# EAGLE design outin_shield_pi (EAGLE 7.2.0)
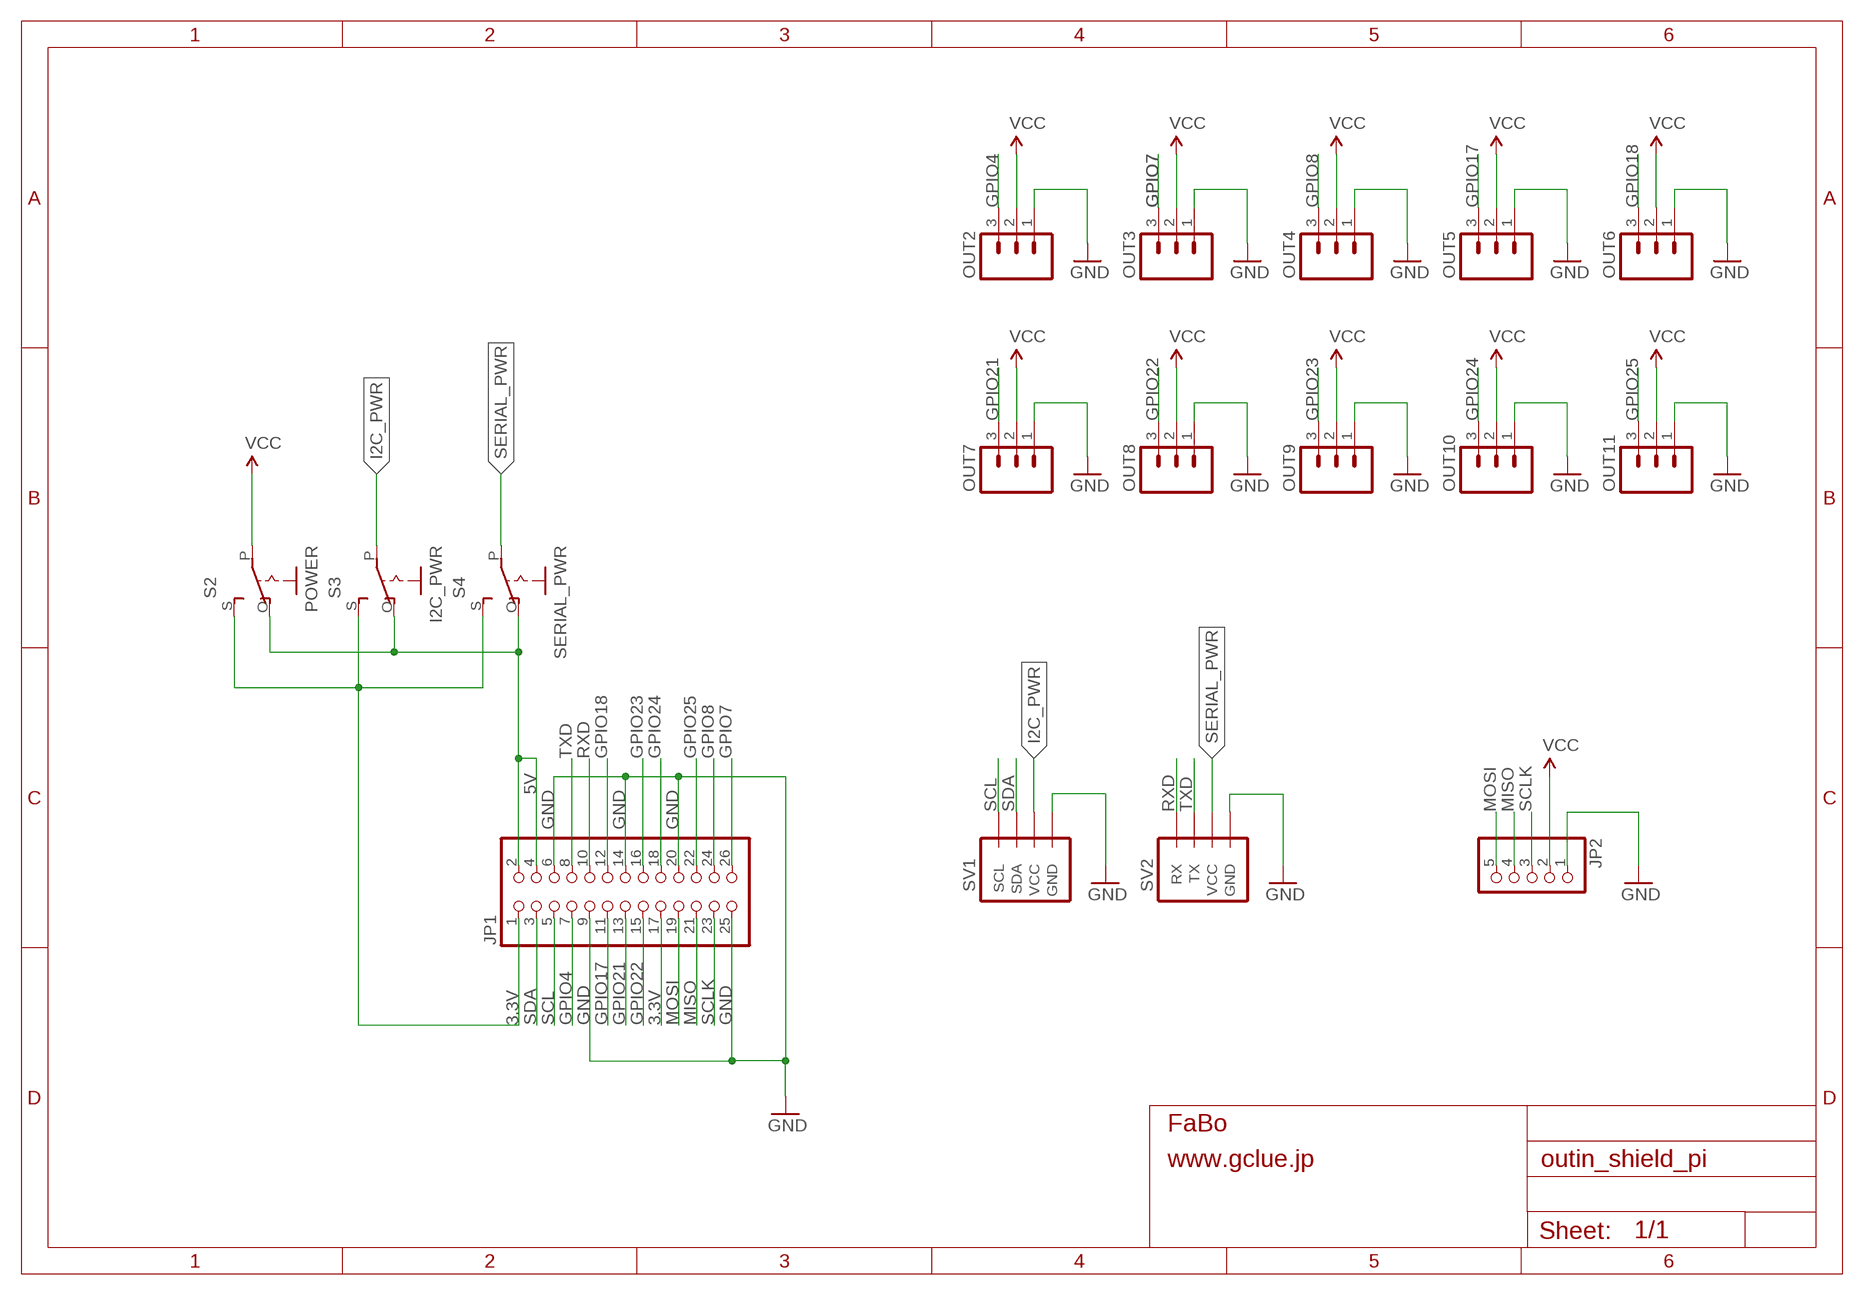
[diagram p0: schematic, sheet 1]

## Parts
JP1  PINHD-2X13  [2X13]
JP2  PINHD-1X5  [1X05]
OUT2  M03PTH  [1X03]
OUT3  M03PTH  [1X03]
OUT4  M03PTH  [1X03]
OUT5  M03PTH  [1X03]
OUT6  M03PTH  [1X03]
OUT7  M03PTH  [1X03]
OUT8  M03PTH  [1X03]
OUT9  M03PTH  [1X03]
OUT10  M03PTH  [1X03]
OUT11  M03PTH  [1X03]
S2  POWER  EG1218S  [EG1218]
S3  I2C_PWR  EG1218S  [EG1218]
S4  SERIAL_PWR  EG1218S  [EG1218]
SV1  BRICK_I2C_CONNECTOR  [BRICK_I2C_CONNECTOR]
SV2  BRICK_SERIAL_CONNECTOR  [BRICK_SERIAL_CONNECTOR]

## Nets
3.3V: JP1.1 JP1.17 S2.S S3.S S4.S
5V: JP1.2 JP1.4 S2.O S3.O S4.O
GND: JP1.6 JP1.9 JP1.14 JP1.20 JP1.25 JP2.1 OUT2.1 OUT3.1 OUT4.1 OUT5.1 OUT6.1 OUT7.1 OUT8.1 OUT9.1 OUT10.1 OUT11.1 SV1.GND SV2.GND
GPIO4: JP1.7 OUT2.3
GPIO7: JP1.26 OUT3.3
GPIO8: JP1.24 OUT4.3
GPIO17: JP1.11 OUT5.3
GPIO18: JP1.12 OUT6.3
GPIO21: JP1.13 OUT7.3
GPIO22: JP1.15 OUT8.3
GPIO23: JP1.16 OUT9.3
GPIO24: JP1.18 OUT10.3
GPIO25: JP1.22 OUT11.3
I2C_PWR: S3.P SV1.VCC
MISO: JP1.21 JP2.4
MOSI: JP1.19 JP2.5
RXD: JP1.10 SV2.RX
SCL: JP1.5 SV1.SCL
SCLK: JP1.23 JP2.3
SDA: JP1.3 SV1.SDA
SERIAL_PWR: S4.P SV2.VCC
TXD: JP1.8 SV2.TX
VCC: JP2.2 OUT2.2 OUT3.2 OUT4.2 OUT5.2 OUT6.2 OUT7.2 OUT8.2 OUT9.2 OUT10.2 OUT11.2 S2.P

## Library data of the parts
JP1 = pinhead:PINHD-2X13: PIN HEADER
JP2 = pinhead:PINHD-1X5: PIN HEADER
OUT2-OUT11 = SparkFun:M03: Header 3 Standard 3-pin 0.1" header. Use with straight break away headers (SKU : PRT-00116), right angle break away headers (PRT-00553), swiss pins (PRT-00743), machine pins (PRT-00117), and female headers (PRT-00115). Molex polarized connector foot print use with SKU : PRT-08232 with associated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
S2-S4 = adafruit:EG1218: SLIDING SWITCH 0.1" spacing through hole, vertical SPDT slide switch http://www.ladyada.net/library/pcb/eaglelibrary.html
SV1 = Gclue:BRICK_I2C_CONNECTOR: Brick Connector female for OUT/IN Shield
SV2 = Gclue:BRICK_SERIAL_CONNECTOR

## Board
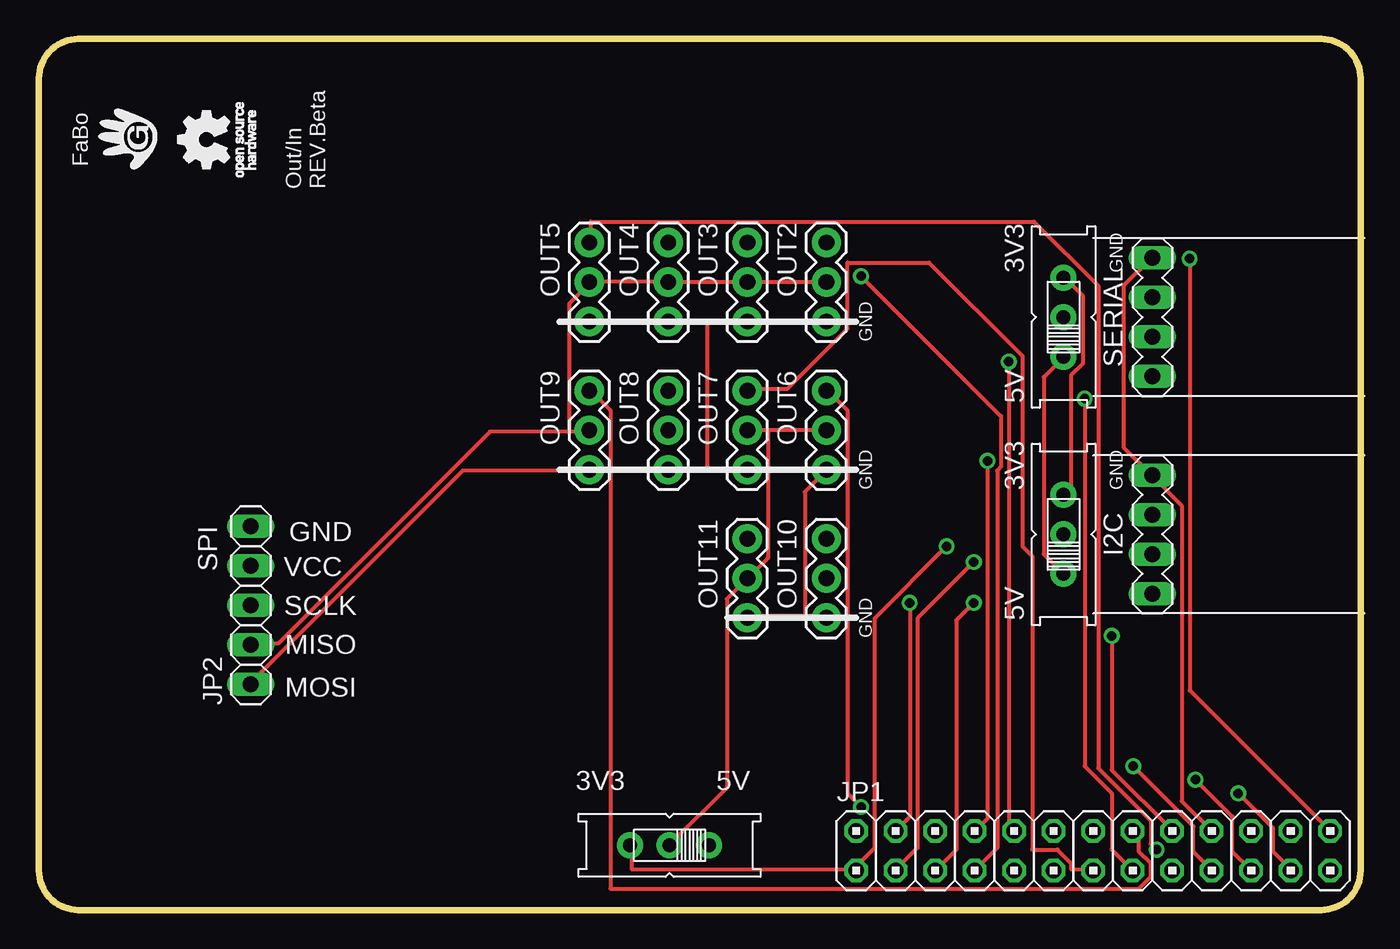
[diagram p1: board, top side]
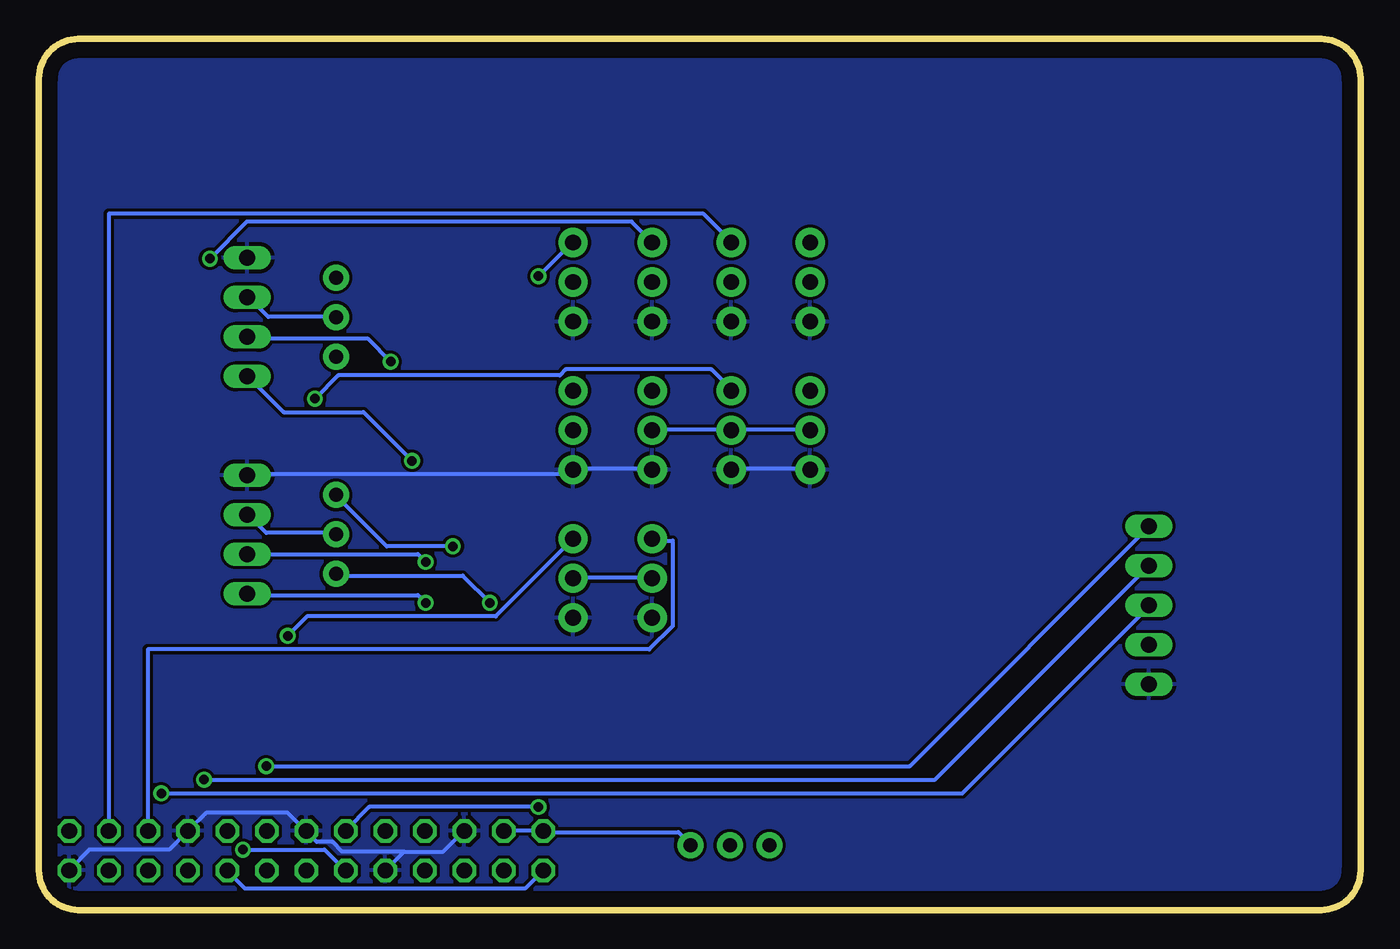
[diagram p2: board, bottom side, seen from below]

Size 85 x 56 mm. Coordinates in mm from the lower left corner, seen from the top.
Outline: 0,53.46 0,2.54 arc90 2.54,0 82.46,0 arc90 85,2.54 85,53.46 arc90 82.46,56 2.54,56 arc90 0,53.46
Copper layers (1*16): Top 0.035mm / dielectric 1.5mm / Bottom 0.035mm
Design rules "default": minimum track width 10mil, minimum drill 24mil, track to track 8mil, track to pad 8mil, pad to pad 8mil, via to via 8mil, smd to smd 8mil, copper to edge 40mil, drill to drill 8mil, minimum pad ring 10mil, minimum via ring 8mil, stop-mask expansion 4mil, vias tented up to drill 0mil, thermal gap 10mil

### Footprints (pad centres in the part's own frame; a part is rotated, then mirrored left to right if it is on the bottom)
2X13 = drill 1.016 octagon: 1 -15.24,-1.27; 2 -15.24,1.27; 3 -12.7,-1.27; 4 -12.7,1.27; 5 -10.16,-1.27; 6 -10.16,1.27; 7 -7.62,-1.27; 8 -7.62,1.27; 9 -5.08,-1.27; 10 -5.08,1.27; 11 -2.54,-1.27; 12 -2.54,1.27; 13 0,-1.27; 14 0,1.27; 15 2.54,-1.27; 16 2.54,1.27; 17 5.08,-1.27; 18 5.08,1.27; 19 7.62,-1.27; 20 7.62,1.27; 21 10.16,-1.27; 22 10.16,1.27; 23 12.7,-1.27; 24 12.7,1.27; 25 15.24,-1.27; 26 15.24,1.27
1X05 = drill 1.016 long: 1 -5.08,0; 2 -2.54,0; 3 0,0; 4 2.54,0; 5 5.08,0
1X03 = drill 1.016 pad 1.88: 1 0,0; 2 2.54,0; 3 5.08,0
EG1218 = drill 0.9 pad 1.676: O -2.54,0; P 0,0; S 2.54,0
BRICK_I2C_CONNECTOR = drill 1.016 long: GND -3.81,0; SCL 3.81,0; SDA 1.27,0; VCC -1.27,0
BRICK_SERIAL_CONNECTOR = drill 1.016 long: GND -3.81,0; RX 1.27,0; TX 3.81,0; VCC -1.27,0

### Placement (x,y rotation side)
JP1  67.8,3.81 0 top
JP2  13.62,19.59 90 top
OUT2  50.64,37.83 90 top
OUT3  45.56,37.83 90 top
OUT4  40.48,37.83 90 top
OUT5  35.4,37.83 90 top
OUT6  50.64,28.3 90 top
OUT7  45.56,28.3 90 top
OUT8  40.48,28.3 90 top
OUT9  35.4,28.3 90 top
OUT10  50.64,18.78 90 top
OUT11  45.56,18.78 90 top
S2  40.56,4.16 180 top
S3  65.89,24.14 90 top
S4  65.89,38.12 90 top
SV1  71.61,24.14 270 top
SV2  71.61,38.12 270 top
U$2  [LOGO_FABO_M]  5.71,49.53 90 top
U$3  [LOGO_OSHW_T_M]  10.79,49.53 90 top

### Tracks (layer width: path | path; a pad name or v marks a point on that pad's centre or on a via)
3.3V  (via drill 0.61)
  Top 0.254: S3.S 66,26.75 66.38,27.12 66.38,34.38 67.12,35.12 67.12,39.5 66,40.62 S4.S | S2.S 38.12,4.12 38.12,2.62 52.5,2.62 JP1.1 52.5,2.75 53.75,4 53.75,18.75 v58.38,23.38
  Bottom 0.254: JP1.17 72.88,2.5 71.75,1.38 53.75,1.38 52.62,2.5 JP1.1 | v58.38,23.38 62.62,23.38 65.88,26.62 S3.S
5V  (via drill 0.61)
  Top 0.254: S3.O 64.62,22.88 64.62,34.25 65.88,35.5 S4.O | v56,19.75 56,6 55.12,5.12 JP1.4
  Bottom 0.254: JP1.4 55,5.12 52.62,5.12 JP1.2 52.5,5 43.88,5 43.12,4.25 S2.O | v56,19.75 57.75,21.5 65.88,21.5 S3.O
GND
  Top 0.254: OUT5.1 35.5,37.88 40.38,37.88 OUT4.1 40.5,37.88 43,37.88 | 43,37.88 45.5,37.88 OUT3.1 45.62,37.88 50.62,37.88 OUT2.1 | SV2.GND 71.5,41.88 69.75,40.12 69.75,29.75 71.5,28 SV1.GND 71.62,27.88 73.5,26 73.5,7 JP1.20 | 49.25,18.88 50.62,18.88 OUT10.1 | 49.25,18.88 45.62,18.88 OUT11.1 | JP2.1 13.62,14.62 27.25,28.25 35.38,28.25 OUT9.1 | 43,28.38 40.5,28.38 OUT8.1 | 43,28.38 45.5,28.38 OUT7.1 | 49.25,18.88 49.25,26.88 50.62,28.25 OUT6.1 | 43,28.38 43,37.88
  Bottom 0.254: 61.5,3.75 59,3.75 57.75,5 JP1.6 | 61.5,3.75 62.62,2.62 JP1.9 | 61.5,3.75 65.5,3.75 66.12,4.38 67.12,4.38 67.75,5 JP1.14 67.88,5.12 69,6.25 74.25,6.25 JP1.20 76.62,3.88 81.75,3.88 83,2.62 JP1.25 | OUT8.1 40.38,28.38 35.5,28.38 OUT9.1 | OUT7.1 45.62,28.38 50.62,28.38 OUT6.1 50.75,28.25 51,28 71.5,28 SV1.GND
  pour Bottom: -1.27,57.15 85.72,57.15 85.72,-0.64 -1.27,-0.64
GPIO4  (via drill 0.61)
  Top 0.254: v52.88,40.75 61.88,31.75 61.88,28.5 61.62,28.25 61.62,4 60.25,2.62 JP1.7
  Bottom 0.254: v52.88,40.75 50.75,42.88 OUT2.3
GPIO7  (via drill 0.61)
  Top 0.254: v74,41.88 74,14.12 83,5.12 JP1.26
  Bottom 0.254: v74,41.88 71.62,44.25 46.88,44.25 45.62,43 OUT3.3
GPIO8
  Bottom 0.254: JP1.24 80.5,44.75 42.25,44.75 40.5,43 OUT4.3
GPIO17  (via drill 0.61)
  Top 0.254: v71.88,3.88 71.5,4.25 71.5,5.75 68.12,9.12 68.12,40.12 64,44.25 35.5,44.25 35.5,43 OUT5.3
  Bottom 0.254: v71.88,3.88 66.62,3.88 65.38,2.62 JP1.11
GPIO18  (via drill 0.61)
  Top 0.254: v52.88,6.62 52,7.5 52,32.12 50.75,33.38 OUT6.3
  Bottom 0.254: v52.88,6.62 63.75,6.62 65.25,5.12 JP1.12
GPIO21
  Top 0.254: JP1.13 67.75,2.62 66.38,2.62 66.38,3 65.5,3.88 63.88,3.88 63.88,22.75 63.25,23.38 63.25,35.62 57.25,41.62 52,41.62 52,37.38 48.12,33.5 45.62,33.5 OUT7.3
GPIO22  (via drill 0.61)
  Top 0.254: v67.25,32.88 67.25,9.25 69,7.5 69,3.88 70.25,2.62 JP1.15
  Bottom 0.254: v67.25,32.88 65.75,34.38 51.5,34.38 51.12,34.75 41.75,34.75 40.5,33.5 OUT8.3
GPIO23
  Top 0.254: JP1.16 70.38,5 70.75,4.62 70.75,3.75 71.5,3 71.5,2.12 70.75,1.38 36.75,1.38 36.75,32.12 35.5,33.38 OUT9.3
GPIO24  (via drill 0.61)
  Top 0.254: v69,17.62 69,9 72.88,5.12 JP1.18
  Bottom 0.254: v69,17.62 67.75,18.88 55.62,18.88 OUT10.3
GPIO25
  Bottom 0.254: JP1.22 78,5.12 78,16.75 45.75,16.75 44.25,18.25 44.25,23.75 45.5,23.75 OUT11.3
I2C_PWR
  Bottom 0.254: SV1.VCC 71.5,25.38 70.38,24.25 66,24.25 S3.P
MISO  (via drill 0.61)
  Top 0.254: v74.38,8.38 76.75,6 76.75,3.75 JP1.21
  Bottom 0.254: JP2.4 27.38,8.38 v74.38,8.38
MOSI  (via drill 0.61)
  Top 0.254: v70.38,9.25 74.25,5.38 74.25,3.75 75.38,2.62 JP1.19
  Bottom 0.254: v70.38,9.25 29,9.25 13.62,24.62 JP2.5
RXD  (via drill 0.61)
  Top 0.254: v62.38,35.25 62.38,5.38 62.62,5.12 JP1.10
  Bottom 0.254: v62.38,35.25 63.88,36.75 71.5,36.75 SV2.RX
SCL  (via drill 0.61)
  Top 0.254: v60.12,19.75 59,18.62 59,3.88 57.75,2.62 JP1.5
  Bottom 0.254: v60.12,19.75 60.62,20.25 71.5,20.25 SV1.SCL
SCLK  (via drill 0.61)
  Top 0.254: v77.12,7.5 79.38,5.25 79.38,3.75 80.5,2.62 JP1.23
  Bottom 0.254: v77.12,7.5 25.62,7.5 13.62,19.5 JP2.3
SDA  (via drill 0.61)
  Top 0.254: v60.12,22.38 56.5,18.75 56.5,4 55.12,2.62 JP1.3
  Bottom 0.254: v60.12,22.38 60.62,22.88 SV1.SDA
SERIAL_PWR
  Bottom 0.254: SV2.VCC 71.5,39.38 70.25,38.12 66,38.12 S4.P
TXD  (via drill 0.61)
  Top 0.254: v61,28.88 61,5.88 60.25,5.12 JP1.8
  Bottom 0.254: v61,28.88 64.12,32 69.25,32 71.5,34.25 SV2.TX
VCC
  Top 0.254: S2.P 40.62,4.25 44.25,7.88 44.25,20 45.5,21.25 OUT11.2 45.62,21.38 46.88,22.62 46.88,30.88 | OUT2.2 50.62,40.38 45.62,40.38 OUT3.2 45.5,40.38 40.5,40.38 OUT4.2 40.38,40.38 35.5,40.38 OUT5.2 35.38,40.25 34.12,39 34.12,30.75 | 34.12,30.75 35.38,30.75 OUT9.2 | 34.12,30.75 29,30.75 15.38,17.12 13.62,17.12 JP2.2 | 46.88,30.88 45.62,30.88 OUT7.2 | 46.88,30.88 50.62,30.88 OUT6.2
  Bottom 0.254: OUT10.2 50.62,21.38 45.62,21.38 OUT11.2 | OUT9.2 35.5,30.88 40.38,30.88 OUT8.2 40.5,30.88 45.5,30.88 OUT7.2

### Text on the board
tPlace: Out/In / REV.Beta | 3V3 | GND | GND | SERIAL | 5V | 3V3 | GND | GND | SPI | GND | I2C | VCC | SCLK | 5V | GND | MISO | MOSI | 3V3 | 5V

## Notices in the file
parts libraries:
SparkFun: Licensing: CC v3.0 Share-Alike You are welcome to use this library for commercial purposes.
